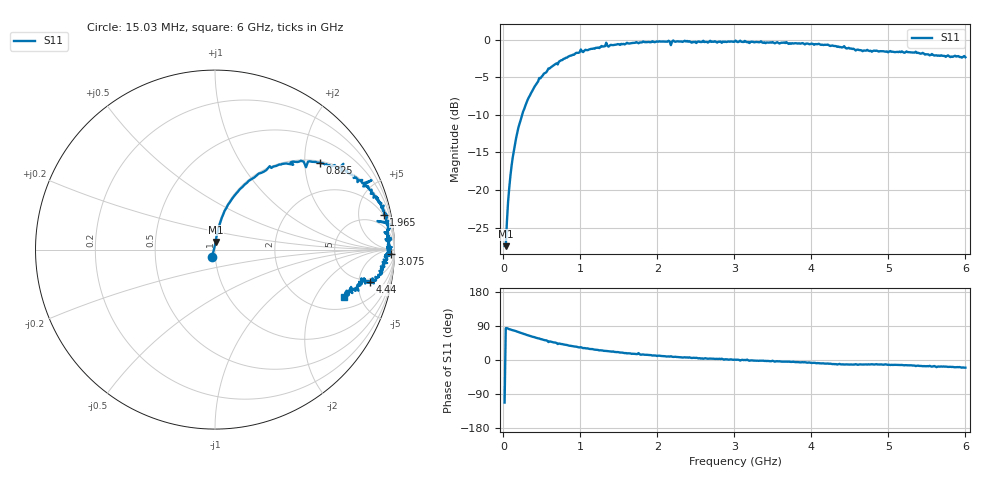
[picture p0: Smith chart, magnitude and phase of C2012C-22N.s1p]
!	Network	Analyzer	HP8753E.07.74:	Oct	30	2002	Serial	No.	JP38451487
!	Hewlett-Packard
!	7	Sep	2009	10:47:45
!	Frequency	S11
#	HZ	S	RI	R	50
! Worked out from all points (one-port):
!   400 points, 15.03 MHz to 6 GHz, reference 50 ohm
!   lowest |S11| = -27.4 dB at 30.03 MHz (marker M1), VSWR 1.09, Z = 50.3 + j4.25 ohm
!   |S11| at or under -10 dB: start of sweep to 242.7 MHz
!   S11 on the Smith chart (normalised r, x): 15.03 MHz: 0.97, -0.08; 825 MHz: 1.05, +2.38; 1.965 GHz: 1.84, +9.40; 3.075 GHz: 35, -54; 4.44 GHz: 4.37, -7.12; 6 GHz: 2.78, -3.51
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1.502992e7  -0.0162 -0.0394
3.002985e7  0.00434 0.0422
6.00297e7  0.0104 0.0828
1.050295e8  0.0264 0.142
1.650292e8  0.0536 0.216
2.550287e8  0.117 0.311
4.650277e8  0.305 0.465
7.650262e8  0.544 0.489
8.250259e8  0.585 0.483
1.335023e9  0.872 0.386
1.365023e9  0.826 0.352
1.515022e9  0.868 0.311
1.755021e9  0.898 0.296
1.785021e9  0.93 0.23
1.96502e9  0.941 0.195
2.145019e9  0.969 0.16
2.175019e9  0.905 0.159
2.205019e9  0.977 0.14
2.265019e9  0.965 0.133
3.015015e9  0.985 0.0138
3.075015e9  0.983 -0.0255
3.165014e9  0.96 0.0167
3.195014e9  0.948 -0.0337
3.765011e9  0.939 -0.077
4.440008e9  0.865 -0.179
4.515007e9  0.855 -0.177
5.265004e9  0.8 -0.201
6e9  0.716 -0.264
